(* Logix 5000 AddOnInstructionDefinition export V430_Copy_Input_4_Decode_104; software revision 33.01 *)

TYPE INPUT_4_Decode_104 :
STRUCT
   Info : V430_InfoBits;
   Device_Status : V430_Device_Status;
   Fault_Code : DINT;
   Counters : V430_CodeReader_Counters;
   Read_Cycle_Report : V430_Read_Cycle_Report;
   Decode1_Report : V430_Decode_Cycle_Report;
   Decode1_Data : V430_4_Decode_160_Char_Str;
   Decode2_Report : V430_Decode_Cycle_Report;
   Decode2_Data : V430_4_Decode_72_Char_Str;
   Decode3_Report : V430_Decode_Cycle_Report;
   Decode3_Data : V430_4_Decode_72_Char_Str;
   Decode4_Report : V430_Decode_Cycle_Report;
   Decode4_Data : V430_4_Decode_72_Char_Str;
END_STRUCT
END_TYPE

TYPE OUTPUT_197 :
STRUCT
   Commands : V430_197_Commands;
END_STRUCT
END_TYPE

TYPE V430_197_Commands :
STRUCT
   Run_Mode : BOOL;
   Trigger : BOOL;
   Enable_Matchcode : BOOL;
   Reset_General_Fault : BOOL;
   Clear_NoRead_ReadCycle_Count : BOOL;
   Clear_MisMatch_ReadCycle_Count : BOOL;
   Clear_NoRead_Count : BOOL;
   Clear_Trigger_Count : BOOL;
   Clear_Matchcode_Count : BOOL;
   Clear_Mismatch_Count : BOOL;
   Output_1 : BOOL;
   Output_2 : BOOL;
   Output_3 : BOOL;
   Reserved1 : BOOL;
   Reserved2 : BOOL;
   Reserved3 : BOOL;
   Reserved4 : BOOL;
   Reserved5 : BOOL;
   Reserved6 : BOOL;
   Reserved7 : BOOL;
   Reserved8 : BOOL;
   Reserved9 : BOOL;
   Reserved10 : BOOL;
   Reserved11 : BOOL;
   Reserved12 : BOOL;
   Reserved13 : BOOL;
   Reserved14 : BOOL;
   Reserved15 : BOOL;
   Reserved16 : BOOL;
   Reserved17 : BOOL;
   Reserved18 : BOOL;
   Reserved19 : BOOL;
END_STRUCT
END_TYPE

TYPE V430_4_Decode_160_Char_Str :   // string type
STRUCT
   LEN : DINT;
   DATA : SINT[160];
END_STRUCT
END_TYPE

TYPE V430_4_Decode_72_Char_Str :   // string type
STRUCT
   LEN : DINT;
   DATA : SINT[72];
END_STRUCT
END_TYPE

TYPE V430_CodeReader_Counters :
STRUCT
   Noread_Read_Cycle_Counter : DINT;
   Mismatch_Per_Read_Cycle_Counter : DINT;
   No_Read_Counter : DINT;
   Trigger_Counter : DINT;
   Match_Code_Counter : DINT;
   Mismatch_Counter : DINT;
END_STRUCT
END_TYPE

TYPE V430_Decode_Cycle_Report :
STRUCT
   Decode_Location_Top : INT;
   Decode_Location_Left : INT;
   Decode_Location_Height : INT;
   Decode_Location_Width : INT;
   Code_Type : V430_Decode_Type;
   Pixels_Per_Element : REAL;
END_STRUCT
END_TYPE

TYPE V430_Decode_Type :
STRUCT
   Aztec : BOOL;
   MicroQR : BOOL;
   Postal_Code : BOOL;
   Code39 : BOOL;
   Codeabar : BOOL;
   I_2of5 : BOOL;
   UPC_EAN : BOOL;
   Code128_EAN128 : BOOL;
   Code93 : BOOL;
   PDF417 : BOOL;
   Pharmacode : BOOL;
   Data_Matrix : BOOL;
   QR_Code : BOOL;
   BC412 : BOOL;
   GS1_Databar : BOOL;
   GS1_Databar_Limited : BOOL;
   GS1_Databar_Expanded : BOOL;
   MicroPDF : BOOL;
   Composite : BOOL;
   Dot_Code : BOOL;
   Reserved_01 : BOOL;
   Reserved_02 : BOOL;
   Reserved_03 : BOOL;
   Reserved_04 : BOOL;
   Reserved_05 : BOOL;
   Reserved_06 : BOOL;
   Reserved_07 : BOOL;
   Reserved_08 : BOOL;
   Reserved_09 : BOOL;
   Reserved_10 : BOOL;
   Reserved_11 : BOOL;
   Reserved_12 : BOOL;
END_STRUCT
END_TYPE

TYPE V430_Device_Status :
STRUCT
   Run_Mode : BOOL;
   Trigger_Ack : BOOL;
   Exposure_Done : BOOL;
   Decoding : BOOL;
   Data_Is_Ready : BOOL;
   Read_Cycle_Pass : BOOL;
   Read_Cycle_Fail : BOOL;
   General_Fault : BOOL;
   New_Matchcode_Ack : BOOL;
   Matchcode_Enabled : BOOL;
   Image_Sensor_Calibrating : BOOL;
   Image_Sensor_Calibrated : BOOL;
   Training : BOOL;
   Train_Completed : BOOL;
   Optimizing : BOOL;
   Optimization_Complete : BOOL;
   Auto_Photometry_Enabled : BOOL;
   Auto_Photometry_Complete : BOOL;
   Output_1_Status : BOOL;
   Output_2_Status : BOOL;
   Output_3_Status : BOOL;
   Buffer_Overflow : BOOL;
   Reserved1 : BOOL;
   Reserved2 : BOOL;
   Reserved3 : BOOL;
   Reserved4 : BOOL; {access Read Only}
   Reserved5 : BOOL; {access Read Only}
   Reserved6 : BOOL; {access Read Only}
   Reserved7 : BOOL; {access Read Only}
   Reserved8 : BOOL; {access Read Only}
   Reserved9 : BOOL; {access Read Only}
   Reserved10 : BOOL; {access Read Only}
END_STRUCT
END_TYPE

TYPE V430_InfoBits :
STRUCT
   InfoBits : SINT;
   Reserved_01 : SINT;
   Reserved_02 : SINT;
   Reserved_03 : SINT;
END_STRUCT
END_TYPE

TYPE V430_Read_Cycle_Report :
STRUCT
   Capture_Time : INT;
   Total_Decode_Time : INT;
   Total_ReadCycle_Time : INT;
   Reserved : INT;
END_STRUCT
END_TYPE

ADD_ON_INSTRUCTION V430_Copy_Input_4_Decode_104   (* revision 1.0, vendor OMRON *)
// Copies Omron V430-F reader EtherNet/IP input and output assemblies to local tags.
// Requires use of Input 4 Decode (104) and Output (197) assemblies.
VAR_IN_OUT
   Assembly_Input : INPUT_4_Decode_104; {required}   // User MicroHAWK Input Assembly
   Assembly_Output : OUTPUT_197; {required}   // User MicroHAWK Output Assembly
   Connection_Input : SINT[500]; {required}   // EIP Input Connection
   Connection_Output : SINT[4]; {required}   // EIP Output Connection
END_VAR

ROUTINE Logic   (* ladder *)
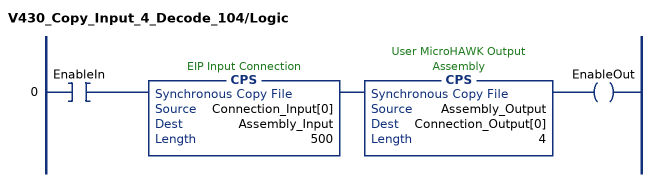
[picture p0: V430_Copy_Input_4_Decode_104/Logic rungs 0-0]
   0: XIC(EnableIn)CPS(Connection_Input[0],Assembly_Input,500)CPS(Assembly_Output,Connection_Output[0],4)OTE(EnableOut);
END_ROUTINE
END_ADD_ON_INSTRUCTION
